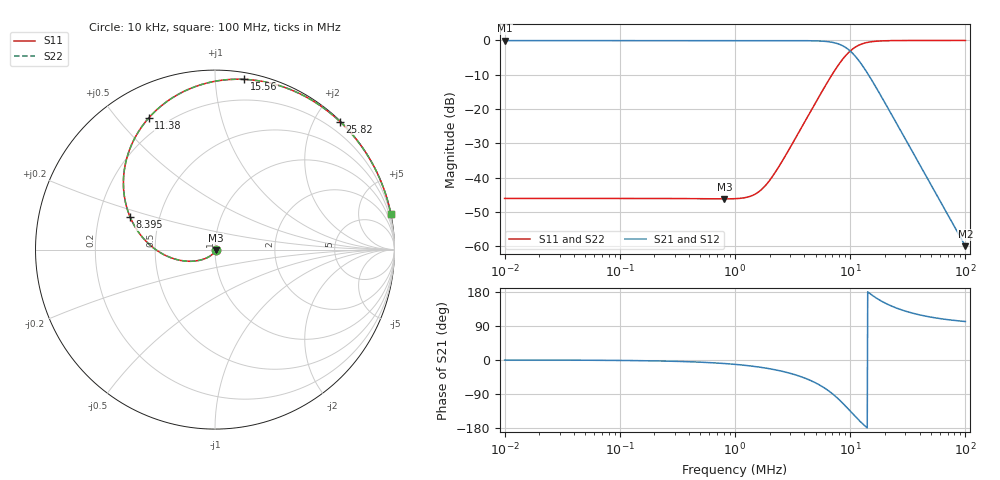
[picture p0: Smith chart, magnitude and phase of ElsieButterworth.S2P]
! 2-port S-parameter file Version 1.0 by Elsie 12/18/2014 5:30:50 PM
# MHz S DB R 50
! Fstart: .01  Fstop: 100  Number of frequencies: 1001
! Freq:  S11 mag:  S11 angle:  S21 mag:  S21 angle:  S12 mag:  S12 angle:  S22 mag:  S22 angle:
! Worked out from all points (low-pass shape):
!   1001 points, 10 kHz to 100 MHz, reference 50 ohm
!   highest |S21| = -0.04 dB at 10 kHz (marker M1); lowest = -60.0 dB at 100 MHz (marker M2)
!   |S21| within 3 dB of the highest: start of sweep to 9.972 MHz
!   lowest |S11| = -46.2 dB at 809.1 kHz (marker M3), VSWR 1.01, Z = 50.5 - j0.132 ohm
!   |S11| at or under -10 dB: start of sweep to 6.952 MHz
!   |S22| runs from -46.2 to 0.0 dB; largest |S21 - S12| = 0
!   S11 on the Smith chart (normalised r, x): 10 kHz: 1.01, -0.00; 8.395 MHz: 0.34, +0.16; 11.38 MHz: 0.13, +0.61; 15.56 MHz: 0.05, +1.18; 25.82 MHz: 0.01, +2.38; 100 MHz: 0.01, +9.95
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0.01  -46.06 -0.1  -0.04 -0.1  -0.04 -0.1  -46.06 -0.1
0.04655861  -46.07 -0.5  -0.04 -0.5  -0.04 -0.5  -46.07 -0.5
0.2167704  -46.09 -2.6  -0.04 -2.5  -0.04 -2.5  -46.09 -2.6
0.8090959  -46.20 -15.4  -0.04 -9.3  -0.04 -9.3  -46.20 -15.4
1  -46.15 -23.1  -0.04 -11.5  -0.04 -11.5  -46.15 -23.1
1.432188  -45.14 -48.3  -0.04 -16.5  -0.04 -16.5  -45.14 -48.3
1.870682  -42.02 -76.7  -0.04 -21.6  -0.04 -21.6  -42.02 -76.7
3.162278  -29.99 -120.0  -0.05 -36.9  -0.05 -36.9  -29.99 -120.0
4.655861  -20.01 -144.3  -0.09 -55.7  -0.09 -55.7  -20.01 -144.3
5.546257  -15.54 -157.2  -0.18 -67.7  -0.18 -67.7  -15.54 -157.2
6.606935  -11.21 -173.0  -0.41 -83.0  -0.41 -83.0  -11.21 -173.0
7.516229  -8.22 173.0  -0.78 -96.8  -0.78 -96.8  -8.22 173.0
8.3946  -5.93 159.2  -1.37 -110.6  -1.37 -110.6  -5.93 159.2
9.817479  -3.33 137.5  -2.85 -132.2  -2.85 -132.2  -3.33 137.5
11.37627  -1.71 116.7  -5.07 -152.9  -5.07 -152.9  -1.71 116.7
13.18257  -0.81 97.9  -8.01 -171.8  -8.01 -171.8  -0.81 97.9
15.55966  -0.33 80.3  -11.85 170.6  -11.85 170.6  -0.33 80.3
18.36538  -0.14 66.3  -15.98 156.6  -15.98 156.6  -0.14 66.3
21.67704  -0.06 55.1  -20.22 145.4  -20.22 145.4  -0.06 55.1
25.8226  -0.03 45.7  -24.75 135.9  -24.75 135.9  -0.03 45.7
44.05549  -0.01 26.2  -38.65 116.4  -38.65 116.4  -0.01 26.2
100  -0.00 11.5  -60.00 101.6  -60.00 101.6  -0.00 11.5
